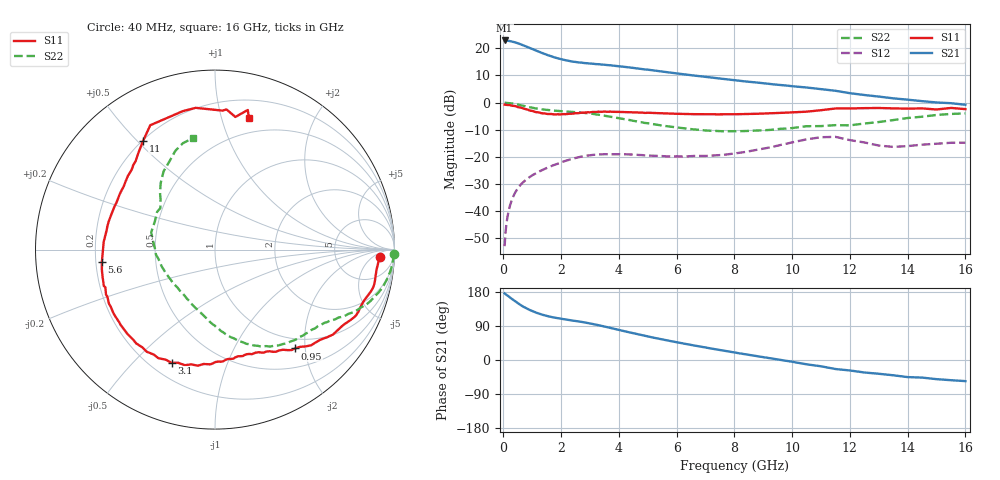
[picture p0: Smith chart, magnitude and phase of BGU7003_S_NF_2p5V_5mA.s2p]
!	Filename:	P:\Prog\Test\Noise\ATS_data\Testdata_Net\BGU7002	BGU7003	RN20082092\BGU7003_B1_high	freq_bias	loop_2.53V4.55mA_D.s2p
!	Date/Time:	Tue	16-Sep-08	9:22:13
!	BGU7003_B1_high	freq_bias	loop
!	bias	mode	1:00	Vout=	2.53	"V,"	Iout=	4.56	"mA,"	Vin=	2.437	"V,"	Iin=	0.473	mA
!	Date/time	Sun	Aug	10	22:27:35	2008
!	Device	data	file	deembeded	for	feedlines	and	parallel
!	Original	file:	\BGU7002	BGU7003	RN20082092\BGU7003_B1_high	freq_bias	loop_2.53V4.55mA_R.s2p
!	Feed-files:	PR029V01_high	"frequency_140808_Feed1.s2p,"	PR029V01_high	frequency_140808_Feed2.s2p
!	Parallel-file:	PR029V01_high	frequency_140808_Par.s2p
#	MHz	S	MA	R	50
!	Freq-MHz	S11-mag	S11-arg	S21-mag	S21-arg	S12-mag	S12-arg	S22-mag	S22-arg
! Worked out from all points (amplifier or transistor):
!   148 points, 40 MHz to 16 GHz, reference 50 ohm
!   highest |S21| = 22.9 dB at 40 MHz (marker M1)
!   |S21| within 3 dB of that: start of sweep to 966.7 MHz
!   unconditionally stable (mu >= 1): nowhere
!   at 280 MHz: K = 0.15, MSG = 29.3 dB, |S12| = -36.2 dB
!   at 1.95 GHz: K = 0.51, MSG = 19.1 dB, |S12| = -22.2 dB
!   at 16 GHz: K = 0.84, MSG = 7.0 dB, |S12| = -14.7 dB
!   lowest NFmin = 0.46 dB at 400 MHz
!   S11 on the Smith chart (normalised r, x): 40 MHz: 19, -10; 950 MHz: 0.82, -1.80; 3.1 GHz: 0.28, -0.65; 5.6 GHz: 0.22, -0.05; 11 GHz: 0.20, +0.52; 16 GHz: 0.35, +1.23
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40  0.9198 -2.5  13.96 175.8  0.00228 80.8  0.9966 -1.4
120  0.9067 -7.9  13.78 171.3  0.00682 83.4  0.9916 -4.4
230  0.9 -14.9  13.57 164.7  0.01295 80.3  0.9783 -8.4
470  0.8389 -29.0  12.54 151.2  0.02508 73.1  0.9291 -16.1
650  0.7924 -38.1  11.56 142.3  0.03304 68.5  0.8854 -20.8
950  0.7085 -51.0  9.953 130.8  0.04419 63.1  0.8174 -26.6
1100  0.6742 -55.9  9.213 125.7  0.04921 60.9  0.786 -28.7
1300  0.6428 -61.7  8.35 120.5  0.05591 58.6  0.7557 -31.4
1500  0.6219 -66.8  7.609 116.2  0.06255 56.5  0.733 -33.9
1700  0.612 -71.8  6.999 112.7  0.06936 54.2  0.7155 -36.4
2150  0.6136 -83.1  6.03 106.8  0.08464 48.4  0.6891 -42.8
2700  0.654 -98.4  5.448 100.6  0.1016 39.2  0.6566 -52.7
3100  0.6757 -111.0  5.204 95.0  0.1093 31.8  0.621 -60.5
4300  0.6684 -146.3  4.486 74.1  0.1117 16.0  0.4849 -81.5
5400  0.6403 -169.9  3.795 55.8  0.1045 11.2  0.3856 -97.1
5600  0.6341 -173.8  3.673 52.8  0.1029 10.9  0.3719 -100.0
6800  0.6136 167.5  3.065 35.7  0.1041 12.8  0.3151 -119.7
8200  0.6141 149.8  2.525 17.3  0.12 18.7  0.2985 -146.1
9600  0.6458 135.6  2.115 0.2  0.1667 16.8  0.3302 -175.1
11000  0.7254 123.6  1.772 -16.6  0.231 -5.0  0.3701 154.8
13500  0.784 93.0  1.2 -40.3  0.1533 -28.9  0.4777 129.3
16000  0.7597 75.6  0.9138 -55.7  0.183 -38.1  0.6333 101.2
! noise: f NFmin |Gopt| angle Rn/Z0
400  0.46  0.42  9.99  0.16
1000  0.58  0.4  25.18  0.16
1500  0.68  0.38  37.84  0.17
1700  0.71  0.38  42.9  0.17
2200  0.81  0.37  55.56  0.16
3000  0.97  0.35  75.81  0.15
4400  1.24  0.34  111.2  0.12
5800  1.51  0.35  146.7  0.1
8000  1.94  0.4  -163.7  0.09
1.2e+04  2.71  0.59  -123.6  0.39
